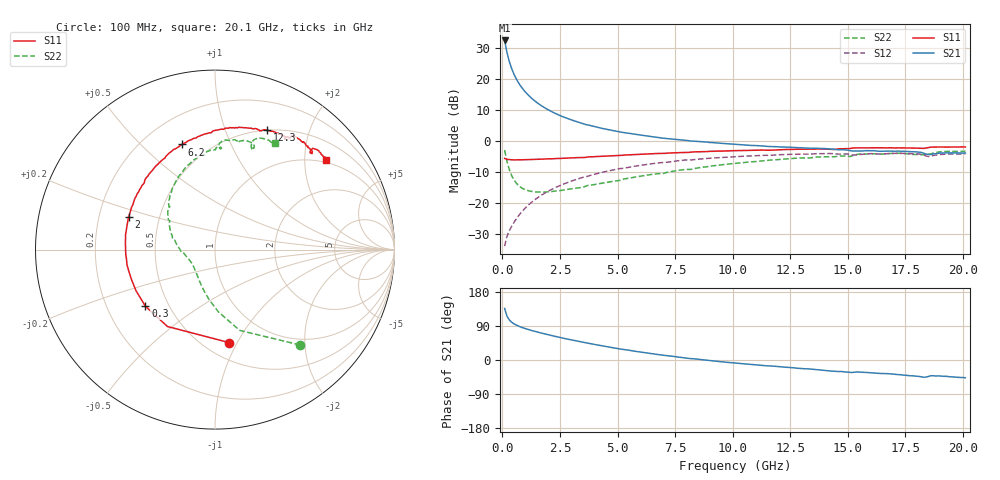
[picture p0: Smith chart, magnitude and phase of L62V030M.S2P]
!  Infineon Technologies AG
! BFR380L3 , PF131585-7, No.6, Th 09.10.01, soldered on pcb-board, measured with PP GSG850
!  Vce=2.0 V,  Ic=30.0 mA
! Common Emitter S-Parameters:  15. November 2001
#  GHz  S  MA  R  50
! f  S11  S21  S12  S22
! GHz  Mag  Ang  Mag  Ang  Mag  Ang  Mag  Ang
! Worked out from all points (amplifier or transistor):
!   201 points, 100 MHz to 20.1 GHz, reference 50 ohm
!   highest |S21| = 32.3 dB at 100 MHz (marker M1)
!   |S21| within 3 dB of that: start of sweep to 179.6 MHz
!   unconditionally stable (mu >= 1): 1.162 GHz to 4.42 GHz
!   at 3.4 GHz: K = 1.02, MAG = 8.1 dB, |S12| = -11.9 dB
!   at 10.1 GHz: K = 0.96, MSG = 2.0 dB, |S12| = -5.1 dB
!   at 20.1 GHz: K = 0.99, MSG = 0.1 dB, |S12| = -4.2 dB
!   S11 on the Smith chart (normalised r, x): 100 MHz: 0.65, -0.92; 300 MHz: 0.37, -0.31; 2 GHz: 0.33, +0.16; 6.2 GHz: 0.36, +0.67; 12.3 GHz: 0.50, +1.41; 20.1 GHz: 0.92, +2.53
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0.1  0.5232 -81.6  41.11 136.2  0.02031 61.1  0.7113 -48.3
0.2  0.5037 -121.7  26.63 116.0  0.02901 55.4  0.4709 -73.0
0.3  0.4999 -140.8  19.04 106.1  0.0357 56.7  0.3469 -87.0
0.4  0.496 -152.4  14.69 100.0  0.04201 58.9  0.2788 -97.0
0.5  0.4943 -159.8  11.91 95.7  0.0485 61.4  0.2376 -104.9
0.6  0.4949 -165.6  10.01 92.4  0.05523 63.0  0.2108 -111.5
0.7  0.4977 -170.2  8.632 89.6  0.06217 64.3  0.1924 -117.3
0.8  0.496 -174.0  7.584 87.1  0.0694 65.3  0.1795 -122.2
1  0.498 180.0  6.114 82.9  0.08354 66.3  0.1637 -130.6
1.3  0.5023 172.6  4.74 77.4  0.1052 66.6  0.1532 -140.2
1.6  0.5068 166.4  3.884 72.5  0.127 66.1  0.1502 -147.6
2  0.5147 159.4  3.146 66.5  0.1558 64.4  0.1517 -155.4
2.6  0.5244 150.0  2.466 58.2  0.1981 61.1  0.161 -164.7
3.5  0.5415 137.2  1.891 46.7  0.2596 55.2  0.1794 -175.3
4.8  0.5769 121.8  1.468 32.4  0.3396 46.1  0.2237 169.2
6.2  0.6138 107.4  1.21 19.1  0.4153 36.1  0.2784 154.7
6.8  0.6274 101.8  1.13 14.0  0.4435 31.7  0.2974 148.3
10.1  0.6963 77.8  0.8805 -8.0  0.5564 10.2  0.4351 120.5
12.3  0.7265 66.4  0.7942 -19.2  0.605 -3.1  0.5133 103.4
13.5  0.7377 60.6  0.7624 -24.4  0.6174 -10.0  0.5412 95.5
16.8  0.7747 48.1  0.6858 -36.4  0.623 -25.5  0.626 75.8
20.1  0.7974 38.9  0.6389 -46.8  0.6174 -38.9  0.681 60.4
